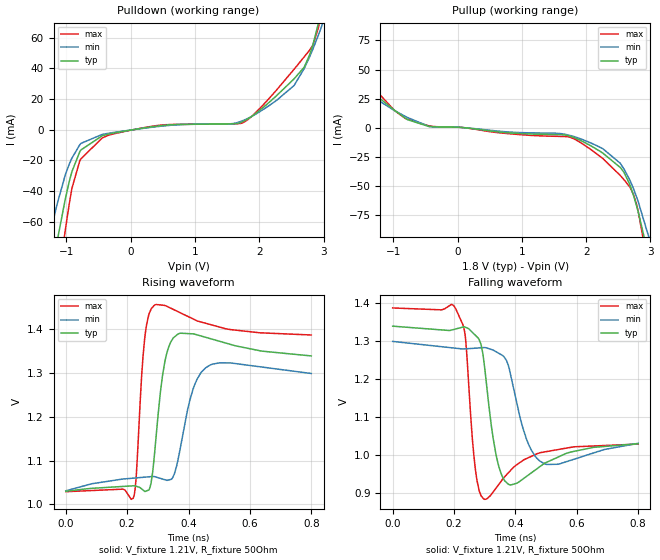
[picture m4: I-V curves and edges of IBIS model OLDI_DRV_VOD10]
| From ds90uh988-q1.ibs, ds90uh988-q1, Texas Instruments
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[Model]   OLDI_DRV_VOD10
Model_type   Output
Polarity   Non-Inverting
Vmeas = 0.55
Vref = 0.55
Cref = 0.02pF
Rref = 50
|   typ   min   max
C_comp   1.47pF   1.46pF   1.53pF
[Voltage Range]   1.8   1.71   1.89
[Temperature Range]   27   105   -40
[Pullup Reference]   1.8   1.71   1.89
[Pulldown Reference]   0   0   0
[Power Clamp Reference]   1.8   1.71   1.89
[GND Clamp Reference]   0   0   0
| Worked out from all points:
|   slope of the pulldown table from 0 to 0.27 V, typ, clamps not added: 151 ohm
|   slope of the pullup table from 0 to 0.27 V, typ, clamps not added: 178 ohm
|   falling waveform, V_fixture 1.21V, R_fixture 50Ohm: 20-80 % time 27.9ps typ, 47.2ps min, 18.4ps max; typ from 1.34 V to 1.03 V
|   rising waveform, V_fixture 1.21V, R_fixture 50Ohm: 20-80 % time 26.2ps typ, 47.4ps min, 16.8ps max; typ from 1.03 V to 1.34 V
[Pulldown]
|   Voltage   I(typ)   I(min)   I(max)
-1.8V     -234.1mA   -175.7mA   -318.1mA
-1.276V   -104.1mA   -72.18mA   -146.6mA
-1.147V   -73.43mA   -48.97mA   -104.9mA
-1.017V   -45.26mA   -29.47mA   -65.46mA
-914.4mV  -27.42mA   -18.57mA   -38.39mA
-774mV    -13.21mA   -8.907mA   -19.01mA
-217.8mV  -1.809mA   -1.496mA   -2.245mA
1.748V    5.346mA    6.005mA    4.609mA
2.542V    33.23mA    28.88mA    39.5mA
2.698V    40.79mA    39.92mA    47.54mA
2.925V    70.43mA    62.37mA    67.61mA
3.6V      242.6mA    147.5mA    430.8mA
[Pullup]
|   Voltage   I(typ)   I(min)   I(max)
-1.8V     86.8mA     75.94mA    75.74mA
-1.66V    54.98mA    57.84mA    59.43mA
-1.568V   43.54mA    46.92mA    51.4mA
-1.346V   31.12mA    27.42mA    36.68mA
-779.4mV  6.823mA    8.67mA     7.115mA
-444.6mV  893.6uA    994.1uA    1.478mA
1.975V    -12.81mA   -11.02mA   -15.17mA
2.531V    -34.39mA   -30.78mA   -41.29mA
2.687V    -50.43mA   -46.21mA   -51.97mA
2.812V    -73.07mA   -64.21mA   -72.78mA
3.006V    -118.8mA   -100.1mA   -132mA
3.6V      -270.7mA   -221.9mA   -333.5mA
[Ramp]
R_load = 50
|   typ   min   max
dV/dt_r   0.185615/2.60196e-11   0.160901/4.70249e-11   0.214925/1.66472e-11
dV/dt_f   0.185615/2.74658e-11   0.160901/4.67458e-11   0.214925/1.83159e-11
[Falling Waveform]
V_fixture = 1.21V
V_fixture_min = 1.21V
V_fixture_max = 1.21V
R_fixture = 50Ohm
C_fixture = 0F
|   Time   V(typ)   V(min)   V(max)
0s        1.339V     1.299V     1.387V
205.2ps   1.332V     1.281V     1.385V
235.2ps   1.337V     1.279V     1.321V
267.9ps   1.316V     1.281V     973.7mV
297.2ps   1.247V     1.283V     884mV
336ps     1.005V     1.272V     911.9mV
377.2ps   923mV      1.235V     953.3mV
424.6ps   936.9mV    1.07V      985.7mV
478.7ps   968.7mV    984.5mV    1.005V
800ps     1.03V      1.031V     1.029V
[Rising Waveform]
V_fixture = 1.21V
V_fixture_min = 1.21V
V_fixture_max = 1.21V
R_fixture = 50Ohm
C_fixture = 0F
|   Time   V(typ)   V(min)   V(max)
0s        1.03V      1.031V     1.029V
219.5ps   1.042V     1.06V      1.014V
229.3ps   1.041V     1.06V      1.062V
256.6ps   1.03V      1.062V     1.376V
288.5ps   1.11V      1.063V     1.455V
322.4ps   1.325V     1.056V     1.454V
365.1ps   1.389V     1.1V       1.44V
414.2ps   1.39V      1.262V     1.424V
455.4ps   1.382V     1.312V     1.414V
800ps     1.339V     1.299V     1.387V
